| IBIS file stm32f302xdxe_303xdxe_lqfp144.ibs
[IBIS ver] 4.2
[File name] stm32f302xdxe_303xdxe_lqfp144.ibs
[File Rev] 1
[Date]  29-09-2025
[Source] Data Created at STMicroelectronics
[Notes]  File originated from ELDO simulations.
[Disclaimer]  This information is for modeling purpose only and is
   not guaranted. The information is subject to change without
   notice.
[Copyright] Copyright 2025 STMicroelectronics Inc.
|   Component stm32f302xdxe_303xdxe_lqfp144
[Component] stm32f302xdxe_303xdxe_lqfp144
[Manufacturer] STMicroelectronics
[Package]
| variable   typ   min   max
R_pkg   0.0   0.0   0.0
L_pkg   0.0H   0.0H   0.0H
C_pkg   0.0F   0.0F   0.0F
[Pin]  signal_name   model_name   R_pin   L_pin   C_pin
1 PE2 io8p_sudq_ft 187.6E-3 9.4E-9 267.9E-15
2 PE3 io8p_sudq_ft 182.4E-3 9.1E-9 243.8E-15
3 PE4 io8p_sudq_ft 177.6E-3 8.7E-9 221.3E-15
4 PE5 io8p_sudq_ft 173.1E-3 8.4E-9 200.2E-15
5 PE6 io8p_sudq_ft 168.9E-3 8.1E-9 180.5E-15
6 VBAT POWER 165.0E-3 7.8E-9 162.3E-15
7 PC13-ANTI-TAMP io8p_sudq_tc 161.5E-3 7.6E-9 145.6E-15
8 PC14-OSC32_IN io8p_sudq_tc 158.2E-3 7.4E-9 130.3E-15
9 PC15-OSC32_OUT io8p_sudq_tc 155.2E-3 7.2E-9 116.4E-15
10 PH0 io8p_sudq_ft 152.6E-3 7.0E-9 104.1E-15
11 PH1 io8p_sudq_ft 150.3E-3 6.8E-9 93.2E-15
12 PF2 io8p_sudq_tc 148.2E-3 6.7E-9 83.7E-15
13 PF3 io8p_sudq_ft 146.5E-3 6.5E-9 75.7E-15
14 PF4 io8p_sudq_tc 145.1E-3 6.4E-9 69.1E-15
15 PF5 io8p_sudq_ft 144.1E-3 6.4E-9 64.0E-15
16 VSS GND 143.3E-3 6.3E-9 60.4E-15
17 VDD POWER 142.8E-3 6.3E-9 58.2E-15
18 PF6 io8p_wsudqh_i2c_ft 142.7E-3 6.3E-9 57.5E-15
19 PF7 io8p_sudq_ft 142.7E-3 6.3E-9 57.5E-15
20 PF8 io8p_sudq_ft 142.8E-3 6.3E-9 58.2E-15
21 PF9 io8p_sudq_ft 143.3E-3 6.3E-9 60.4E-15
22 PF10 io8p_sudq_ft 144.1E-3 6.4E-9 64.0E-15
23 PF0-OSC_IN io8p_wsudqh_i2c_ft 145.1E-3 6.4E-9 69.1E-15
24 PF1-OSC_OUT io8p_wsudqh_i2c_ft 146.5E-3 6.5E-9 75.7E-15
25 NRST ioreset_tc_v33 148.2E-3 6.7E-9 83.7E-15
26 PC0 io8p_sudq_tc 150.3E-3 6.8E-9 93.2E-15
27 PC1 io8p_sudq_tc 152.6E-3 7.0E-9 104.1E-15
28 PC2 io8p_sudq_tc 155.2E-3 7.2E-9 116.4E-15
29 PC3 io8p_sudq_tc 158.2E-3 7.4E-9 130.3E-15
30 VSSA GND 161.5E-3 7.6E-9 145.6E-15
31 VREF- GND 165.0E-3 7.8E-9 162.3E-15
32 VREF+ POWER 168.9E-3 8.1E-9 180.5E-15
33 VDDA POWER 173.1E-3 8.4E-9 200.2E-15
34 PA0-WKUP io8p_sudq_tc 177.6E-3 8.7E-9 221.3E-15
35 PA1 io8p_sudq_tc 182.4E-3 9.1E-9 243.8E-15
36 PA2 io8p_sudq_tc 187.6E-3 9.4E-9 267.9E-15
37 PA3 io8p_sudq_tc 187.6E-3 9.4E-9 267.9E-15
38 VSS GND 182.4E-3 9.1E-9 243.8E-15
39 VDD POWER 177.6E-3 8.7E-9 221.3E-15
40 PA4 io8p_sudq_tc 173.1E-3 8.4E-9 200.2E-15
41 PA5 io8p_sudq_tc 168.9E-3 8.1E-9 180.5E-15
42 PA6 io8p_sudq_tc 165.0E-3 7.8E-9 162.3E-15
43 PA7 io8p_sudq_tc 161.5E-3 7.6E-9 145.6E-15
44 PC4 io8p_sudq_tc 158.2E-3 7.4E-9 130.3E-15
45 PC5 io8p_sudq_tc 155.2E-3 7.2E-9 116.4E-15
46 PB0 io8p_sudq_tc 152.6E-3 7.0E-9 104.1E-15
47 PB1 io8p_sudq_tc 150.3E-3 6.8E-9 93.2E-15
48 PB2 io8p_sudq_tc 148.2E-3 6.7E-9 83.7E-15
49 PF11 io8p_sudq_ft 146.5E-3 6.5E-9 75.7E-15
50 PF12 io8p_sudq_ft 145.1E-3 6.4E-9 69.1E-15
51 VSS GND 144.1E-3 6.4E-9 64.0E-15
52 VDD POWER 143.3E-3 6.3E-9 60.4E-15
53 PF13 io8p_sudq_ft 142.8E-3 6.3E-9 58.2E-15
54 PF14 io8p_sudq_ft 142.7E-3 6.3E-9 57.5E-15
55 PF15 io8p_sudq_ft 142.7E-3 6.3E-9 57.5E-15
56 PG0 io8p_sudq_ft 142.8E-3 6.3E-9 58.2E-15
57 PG1 io8p_sudq_ft 143.3E-3 6.3E-9 60.4E-15
58 PE7 io8p_sudq_tc 144.1E-3 6.4E-9 64.0E-15
59 PE8 io8p_sudq_tc 145.1E-3 6.4E-9 69.1E-15
60 PE9 io8p_sudq_tc 146.5E-3 6.5E-9 75.7E-15
61 VSS GND 148.2E-3 6.7E-9 83.7E-15
62 VDD POWER 150.3E-3 6.8E-9 93.2E-15
63 PE10 io8p_sudq_tc 152.6E-3 7.0E-9 104.1E-15
64 PE11 io8p_sudq_tc 155.2E-3 7.2E-9 116.4E-15
65 PE12 io8p_sudq_tc 158.2E-3 7.4E-9 130.3E-15
66 PE13 io8p_sudq_tc 161.5E-3 7.6E-9 145.6E-15
67 PE14 io8p_sudq_tc 165.0E-3 7.8E-9 162.3E-15
68 PE15 io8p_sudq_tc 168.9E-3 8.1E-9 180.5E-15
69 PB10 io8p_sudq_tc 173.1E-3 8.4E-9 200.2E-15
70 PB11 io8p_sudq_tc 177.6E-3 8.7E-9 221.3E-15
71 VSS GND 182.4E-3 9.1E-9 243.8E-15
72 VDD POWER 187.6E-3 9.4E-9 267.9E-15
73 PB12 io8p_sudq_tc 187.6E-3 9.4E-9 267.9E-15
74 PB13 io8p_sudq_tc 182.4E-3 9.1E-9 243.8E-15
75 PB14 io8p_sudq_tc 177.6E-3 8.7E-9 221.3E-15
76 PB15 io8p_sudq_tc 173.1E-3 8.4E-9 200.2E-15
77 PD8 io8p_sudq_tc 168.9E-3 8.1E-9 180.5E-15
78 PD9 io8p_sudq_tc 165.0E-3 7.8E-9 162.3E-15
79 PD10 io8p_sudq_tc 161.5E-3 7.6E-9 145.6E-15
80 PD11 io8p_sudq_tc 158.2E-3 7.4E-9 130.3E-15
81 PD12 io8p_sudq_tc 155.2E-3 7.2E-9 116.4E-15
82 PD13 io8p_sudq_tc 152.6E-3 7.0E-9 104.1E-15
83 VSS GND 150.3E-3 6.8E-9 93.2E-15
84 VDD POWER 148.2E-3 6.7E-9 83.7E-15
85 PD14 io8p_sudq_tc 146.5E-3 6.5E-9 75.7E-15
86 PD15 io8p_sudq_tc 145.1E-3 6.4E-9 69.1E-15
87 PG2 io8p_sudq_ft 144.1E-3 6.4E-9 64.0E-15
88 PG3 io8p_sudq_ft 143.3E-3 6.3E-9 60.4E-15
89 PG4 io8p_sudq_ft 142.8E-3 6.3E-9 58.2E-15
90 PG5 io8p_sudq_ft 142.7E-3 6.3E-9 57.5E-15
91 PG6 io8p_sudq_ft 142.7E-3 6.3E-9 57.5E-15
92 PG7 io8p_sudq_ft 142.8E-3 6.3E-9 58.2E-15
93 PG8 io8p_sudq_ft 143.3E-3 6.3E-9 60.4E-15
94 VSS GND 144.1E-3 6.4E-9 64.0E-15
95 VDD POWER 145.1E-3 6.4E-9 69.1E-15
96 PC6 io8p_sudq_ft 146.5E-3 6.5E-9 75.7E-15
97 PC7 io8p_sudq_ft 148.2E-3 6.7E-9 83.7E-15
98 PC8 io8p_sudq_ft 150.3E-3 6.8E-9 93.2E-15
99 PC9 io8p_wsudqh_i2c_ft 152.6E-3 7.0E-9 104.1E-15
100 PA8 io8p_wsudqh_i2c_ft 155.2E-3 7.2E-9 116.4E-15
101 PA9 io8p_wsudqh_i2c_ft 158.2E-3 7.4E-9 130.3E-15
102 PA10 io8p_wsudqh_i2c_ft 161.5E-3 7.6E-9 145.6E-15
103 PA11 io8usb_lv_ft 165.0E-3 7.8E-9 162.3E-15
104 PA12 io8usb_lv_ft 168.9E-3 8.1E-9 180.5E-15
105 PA13 io8p_wsudqh_i2c_ft 173.1E-3 8.4E-9 200.2E-15
106 PH2 io8p_sudq_ft 177.6E-3 8.7E-9 221.3E-15
107 VSS GND 182.4E-3 9.1E-9 243.8E-15
108 VDD POWER 187.6E-3 9.4E-9 267.9E-15
109 PA14 io8p_wsudqh_i2c_ft 187.6E-3 9.4E-9 267.9E-15
110 PA15 io8p_wsudqh_i2c_ft 182.4E-3 9.1E-9 243.8E-15
111 PC10 io8p_sudq_ft 177.6E-3 8.7E-9 221.3E-15
112 PC11 io8p_sudq_ft 173.1E-3 8.4E-9 200.2E-15
113 PC12 io8p_sudq_ft 168.9E-3 8.1E-9 180.5E-15
114 PD0 io8p_sudq_ft 165.0E-3 7.8E-9 162.3E-15
115 PD1 io8p_sudq_ft 161.5E-3 7.6E-9 145.6E-15
116 PD2 io8p_sudq_ft 158.2E-3 7.4E-9 130.3E-15
117 PD3 io8p_sudq_ft 155.2E-3 7.2E-9 116.4E-15
118 PD4 io8p_sudq_ft 152.6E-3 7.0E-9 104.1E-15
119 PD5 io8p_sudq_ft 150.3E-3 6.8E-9 93.2E-15
120 VSS GND 148.2E-3 6.7E-9 83.7E-15
121 VDD POWER 146.5E-3 6.5E-9 75.7E-15
122 PD6 io8p_sudq_ft 145.1E-3 6.4E-9 69.1E-15
123 PD7 io8p_sudq_ft 144.1E-3 6.4E-9 64.0E-15
124 PG9 io8p_sudq_ft 143.3E-3 6.3E-9 60.4E-15
125 PG10 io8p_sudq_ft 142.8E-3 6.3E-9 58.2E-15
126 PG11 io8p_sudq_ft 142.7E-3 6.3E-9 57.5E-15
127 PG12 io8p_sudq_ft 142.7E-3 6.3E-9 57.5E-15
128 PG13 io8p_sudq_ft 142.8E-3 6.3E-9 58.2E-15
129 PG14 io8p_sudq_ft 143.3E-3 6.3E-9 60.4E-15
130 VSS GND 144.1E-3 6.4E-9 64.0E-15
131 VDD POWER 145.1E-3 6.4E-9 69.1E-15
132 PG15 io8p_sudq_ft 146.5E-3 6.5E-9 75.7E-15
133 PB3 io8p_sudq_ft 148.2E-3 6.7E-9 83.7E-15
134 PB4 io8p_sudq_ft 150.3E-3 6.8E-9 93.2E-15
135 PB5 io8p_wsudqh_i2c_ft 152.6E-3 7.0E-9 104.1E-15
136 PB6 io8p_wsudqh_i2c_ft 155.2E-3 7.2E-9 116.4E-15
137 PB7 io8p_wsudqh_i2c_ft 158.2E-3 7.4E-9 130.3E-15
138 BOOT0 vpp_test_hv 161.5E-3 7.6E-9 145.6E-15
139 PB8 io8p_wsudqh_i2c_ft 165.0E-3 7.8E-9 162.3E-15
140 PB9 io8p_wsudqh_i2c_ft 168.9E-3 8.1E-9 180.5E-15
141 PE0 io8p_sudq_ft 173.1E-3 8.4E-9 200.2E-15
142 PE1 io8p_sudq_ft 177.6E-3 8.7E-9 221.3E-15
143 VSS GND 182.4E-3 9.1E-9 243.8E-15
144 VDD POWER 187.6E-3 9.4E-9 267.9E-15
[Model Selector] io8p_sudq_ft
io8p01_sudq_ft_pd_lv  "SPEED01 2P0V, PD=40kOhm"
io8p01_sudq_ft_pu_lv  "SPEED01 2P0V, PU=40kOhm"
io8p01_sudq_ft_lv  "SPEED01 2P0V"
io8p10_sudq_ft_pd_lv  "SPEED10 2P0V, PD=40kOhm"
io8p10_sudq_ft_pu_lv  "SPEED10 2P0V, PU=40kOhm"
io8p10_sudq_ft_lv  "SPEED10 2P0V"
io8p11_sudq_ft_pd_lv  "SPEED11 2P0V, PD=40kOhm"
io8p11_sudq_ft_pu_lv  "SPEED11 2P0V, PU=40kOhm"
io8p11_sudq_ft_lv  "SPEED11 2P0V"
io8p01_sudq_ft_pd  "SPEED01, PD=40kOhm"
io8p01_sudq_ft_pu  "SPEED01, PU=40kOhm"
io8p01_sudq_ft  "SPEED01"
io8p10_sudq_ft_pd  "SPEED10, PD=40kOhm"
io8p10_sudq_ft_pu  "SPEED10, PU=40kOhm"
io8p10_sudq_ft  "SPEED10"
io8p11_sudq_ft_pd  "SPEED11, PD=40kOhm"
io8p11_sudq_ft_pu  "SPEED11, PU=40kOhm"
io8p11_sudq_ft  "SPEED11"
[Model Selector] io8p_sudq_tc
io8p01_sudq_tc_pd_lv  "SPEED01 2P0V, PD=40kOhm"
io8p01_sudq_tc_pu_lv  "SPEED01 2P0V, PU=40kOhm"
io8p01_sudq_tc_lv  "SPEED01 2P0V"
io8p10_sudq_tc_pd_lv  "SPEED10 2P0V, PD=40kOhm"
io8p10_sudq_tc_pu_lv  "SPEED10 2P0V, PU=40kOhm"
io8p10_sudq_tc_lv  "SPEED10 2P0V"
io8p11_sudq_tc_pd_lv  "SPEED11 2P0V, PD=40kOhm"
io8p11_sudq_tc_pu_lv  "SPEED11 2P0V, PU=40kOhm"
io8p11_sudq_tc_lv  "SPEED11 2P0V"
io8p01_sudq_tc_pd  "SPEED01, PD=40kOhm"
io8p01_sudq_tc_pu  "SPEED01, PU=40kOhm"
io8p01_sudq_tc  "SPEED01"
io8p10_sudq_tc_pd  "SPEED10, PD=40kOhm"
io8p10_sudq_tc_pu  "SPEED10, PU=40kOhm"
io8p10_sudq_tc  "SPEED10"
io8p11_sudq_tc_pd  "SPEED11, PD=40kOhm"
io8p11_sudq_tc_pu  "SPEED11, PU=40kOhm"
io8p11_sudq_tc  "SPEED11"
[Model Selector] io8p_wsudqh_i2c_ft
io8p_wsudqh_i2c_ft_lv_pd  "General purpose IO with I2C capability on. 5V tolerant. 1.8V range with pull down"
io8p_wsudqh_i2c_ft_lv_pu  "General purpose IO with I2C capability on. 5V tolerant. 1.8V range with pull up"
io8p_wsudqh_i2c_ft_lv  "General purpose IO with I2C capability on. 5V tolerant. 1.8V range"
io8p_wsudqh_i2c_ft_pd  "General purpose IO with I2C capability on. 5V tolerant. 3.3V range with pull down"
io8p_wsudqh_i2c_ft_pu  "General purpose IO with I2C capability on. 5V tolerant. 3.3V range with pull up"
io8p_wsudqh_i2c_ft_i2c  "General purpose IO with I2C capability on. 5V tolerant. 3.3V range"
[Model Selector] io8usb_lv_ft
io8usb_dpdn_lv_ft_pd  "FS USB DP/DN IO + PD=40kOhm"
io8usb_dpdn_lv_ft_pu  "FS USB DP/DN IO + PU=40kOhm"
io8usb_dpdn_lv_ft  "FS USB DP/DN IO"
io8p01_lv_ft_pd_lv  "SPEED01 2P0V, PD=40kOhm"
io8p01_lv_ft_pu_lv  "SPEED01 2P0V, PU=40kOhm"
io8p01_lv_ft_lv  "SPEED01 2P0V"
io8p10_lv_ft_pd_lv  "SPEED10 2P0V, PD=40kOhm"
io8p10_lv_ft_pu_lv  "SPEED10 2P0V, PU=40kOhm"
io8p10_lv_ft_lv  "SPEED10 2P0V"
io8p11_lv_ft_pd_lv  "SPEED11 2P0V, PD=40kOhm"
io8p11_lv_ft_pu_lv  "SPEED11 2P0V, PU=40kOhm"
io8p11_lv_ft_lv  "SPEED11 2P0V"
io8p01_lv_ft_pd  "SPEED01, PD=40kOhm"
io8p01_lv_ft_pu  "SPEED01, PU=40kOhm"
io8p01_lv_ft  "SPEED01"
io8p10_lv_ft_pd  "SPEED10, PD=40kOhm"
io8p10_lv_ft_pu  "SPEED10, PU=40kOhm"
io8p10_lv_ft  "SPEED10"
io8p11_lv_ft_pd  "SPEED11, PD=40kOhm"
io8p11_lv_ft_pu  "SPEED11, PU=40kOhm"
io8p11_lv_ft  "SPEED11"
[Model Selector] ioreset_tc_v33
ioreset_tc_v33_pu_lv  "IORESET 2V + PU=40kOhm"
ioreset_tc_v33_nopu_lv  "IORESET 2V"
ioreset_tc_v33_pu  "IORESET + PU=40kOhm"
ioreset_tc_v33_nopu  "IORESET"
[Model Selector] vpp_test_hv
vpp_test_hv_3p3  "Input Buffer"
vpp_test_hv_2p4  "Input Buffer 2P0V"
| Models and submodels in the file (69): io8p01_sudq_ft_pd_lv (I/O), io8p01_sudq_ft_pu_lv (I/O), io8p01_sudq_ft_lv (I/O), io8p10_sudq_ft_pd_lv (I/O), io8p10_sudq_ft_pu_lv (I/O), io8p10_sudq_ft_lv (I/O), io8p11_sudq_ft_pd_lv (I/O), io8p11_sudq_ft_pu_lv (I/O), io8p11_sudq_ft_lv (I/O), io8p01_sudq_ft_pd (I/O), io8p01_sudq_ft_pu (I/O), io8p01_sudq_ft (I/O), io8p10_sudq_ft_pd (I/O), io8p10_sudq_ft_pu (I/O), io8p10_sudq_ft (I/O), io8p11_sudq_ft_pd (I/O), io8p11_sudq_ft_pu (I/O), io8p11_sudq_ft (I/O), io8p01_sudq_tc_pd_lv (I/O), io8p01_sudq_tc_pu_lv (I/O), io8p01_sudq_tc_lv (I/O), io8p10_sudq_tc_pd_lv (I/O), io8p10_sudq_tc_pu_lv (I/O), io8p10_sudq_tc_lv (I/O), io8p11_sudq_tc_pd_lv (I/O), io8p11_sudq_tc_pu_lv (I/O), io8p11_sudq_tc_lv (I/O), io8p01_sudq_tc_pd (I/O), io8p01_sudq_tc_pu (I/O), io8p01_sudq_tc (I/O), io8p10_sudq_tc_pd (I/O), io8p10_sudq_tc_pu (I/O), io8p10_sudq_tc (I/O), io8p11_sudq_tc_pd (I/O), io8p11_sudq_tc_pu (I/O), io8p11_sudq_tc (I/O), io8p_wsudqh_i2c_ft_lv_pd (I/O), io8p_wsudqh_i2c_ft_lv_pu (I/O), io8p_wsudqh_i2c_ft_lv (I/O), io8p_wsudqh_i2c_ft_pd (I/O), io8p_wsudqh_i2c_ft_pu (I/O), io8p_wsudqh_i2c_ft_i2c (I/O), io8usb_dpdn_lv_ft_pd (I/O), io8usb_dpdn_lv_ft_pu (I/O), io8usb_dpdn_lv_ft (I/O), io8p01_lv_ft_pd_lv (I/O), io8p01_lv_ft_pu_lv (I/O), io8p01_lv_ft_lv (I/O), io8p10_lv_ft_pd_lv (I/O), io8p10_lv_ft_pu_lv (I/O), io8p10_lv_ft_lv (I/O), io8p11_lv_ft_pd_lv (I/O), io8p11_lv_ft_pu_lv (I/O), io8p11_lv_ft_lv (I/O), io8p01_lv_ft_pd (I/O), io8p01_lv_ft_pu (I/O), io8p01_lv_ft (I/O), io8p10_lv_ft_pd (I/O), io8p10_lv_ft_pu (I/O), io8p10_lv_ft (I/O), io8p11_lv_ft_pd (I/O), io8p11_lv_ft_pu (I/O), io8p11_lv_ft (I/O), ioreset_tc_v33_pu_lv (I/O_open_drain), ioreset_tc_v33_nopu_lv (I/O_open_drain), ioreset_tc_v33_pu (I/O_open_drain), ioreset_tc_v33_nopu (I/O_open_drain), vpp_test_hv_2p4 (Input), vpp_test_hv_3p3 (Input)
